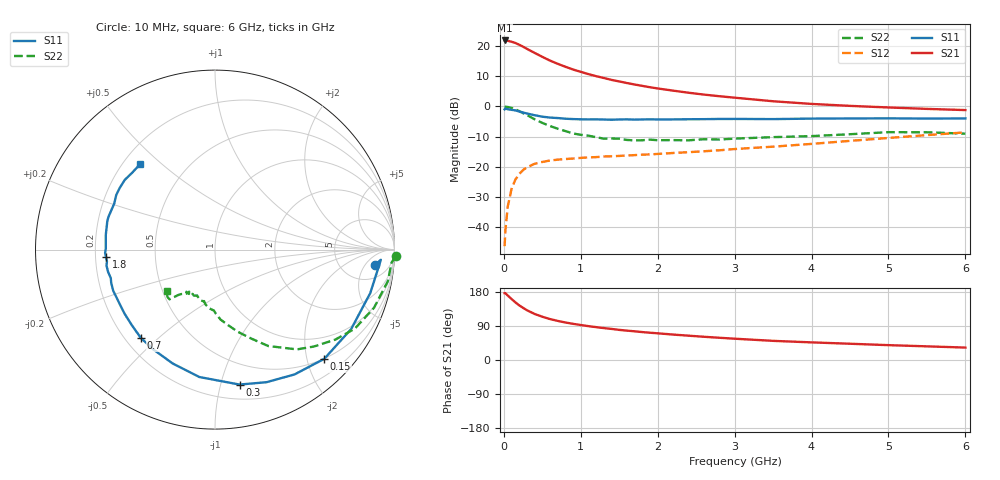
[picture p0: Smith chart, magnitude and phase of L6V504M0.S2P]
!  INFINEON TECHNOLOGIES Small Signal Semiconductors
! BFR380L3 , Si-NPN RF-Transistor in TSLP-3-1
!  Vce=0.5 V,  Ic=4 mA
! Common Emitter S-Parameters:  07. March 2005
#  GHz  S  MA  R  50
! f  S11  S21  S12  S22
! GHz  Mag  Ang  Mag  Ang  Mag  Ang  Mag  Ang
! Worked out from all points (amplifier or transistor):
!   36 points, 10 MHz to 6 GHz, reference 50 ohm
!   highest |S21| = 21.8 dB at 10 MHz (marker M1)
!   |S21| within 3 dB of that: start of sweep to 317.3 MHz
!   unconditionally stable (mu >= 1): 2.291 GHz to 5.339 GHz
!   at 250 MHz: K = 0.16, MSG = 20.4 dB, |S12| = -21.0 dB
!   at 1.4 GHz: K = 0.75, MSG = 12.6 dB, |S12| = -16.5 dB
!   at 6 GHz: K = 0.99, MSG = 3.7 dB, |S12| = -8.6 dB
!   S11 on the Smith chart (normalised r, x): 10 MHz: 10, -9; 150 MHz: 0.49, -2.32; 300 MHz: 0.32, -1.15; 700 MHz: 0.26, -0.44; 1.8 GHz: 0.24, -0.03; 6 GHz: 0.27, +0.43
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0.01  0.8938 -5.6  12.31 176.4  0.0049 81.3  1.008 -2.1
0.02  0.9259 -3.5  12.26 176.5  0.0088 92.6  0.9864 -4.2
0.05  0.8985 -15.6  12.18 170.2  0.0219 82.5  0.9792 -10.3
0.1  0.8784 -30.2  11.71 161.0  0.0432 74.7  0.9435 -20.1
0.15  0.8608 -45.0  11.19 152.1  0.0618 66.0  0.8949 -29.5
0.2  0.8247 -57.5  10.45 144.2  0.0764 60.5  0.8371 -36.8
0.25  0.7925 -68.8  9.712 137.6  0.0888 55.2  0.7717 -44.4
0.3  0.7642 -79.7  8.951 131.4  0.0986 50.9  0.7195 -50.6
0.4  0.7152 -97.0  7.668 121.5  0.1125 44.2  0.6135 -61.1
0.5  0.6769 -110.4  6.598 114.2  0.1209 40.0  0.5337 -68.0
0.6  0.654 -121.6  5.722 108.0  0.1275 37.0  0.4749 -74.5
0.7  0.6426 -130.0  5.064 103.2  0.1319 35.4  0.4277 -80.1
0.9  0.6177 -144.5  4.075 95.4  0.1377 33.4  0.357 -89.2
1.1  0.6101 -153.8  3.42 89.3  0.1437 33.4  0.3287 -95.7
1.4  0.6019 -164.7  2.746 82.0  0.15 34.1  0.2954 -103.2
1.8  0.609 -176.3  2.186 73.7  0.1594 36.9  0.2758 -111.9
2.2  0.6101 175.7  1.824 67.1  0.1699 40.1  0.2775 -116.6
2.8  0.6205 165.3  1.475 58.7  0.1883 45.3  0.2837 -124.1
3.5  0.6173 155.5  1.217 50.5  0.2161 49.1  0.3107 -127.1
4.5  0.6323 147.2  1.021 42.9  0.2696 53.9  0.3471 -130.6
5.5  0.6296 136.9  0.91 36.0  0.3356 54.4  0.3736 -135.2
6  0.6331 131.1  0.87 32.8  0.3727 53.5  0.3544 -139.6
